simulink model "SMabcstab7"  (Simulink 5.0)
settings: Solver=ode45  StartTime=0.0  StopTime=6  MaxStep=2e-4  RelTol=1e-4
InitFcn:
  | smparamstab7
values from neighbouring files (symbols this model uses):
  Bm = 0.10    (= 0.1)    [IMabc2.m]    (also in imabcparam.m = 0.01; IMabcrun0.m = 0.01; IMabcrun1.m = 0.001; IMcur0.m = 1e-06)
  gam = 2*pi/3    (= 2.09439510239)    [IMabc2.m]    (also in IMabcf0.m; IMabcf1.m; imabcparam.m; IMabcrun0.m)
  H = 0.60    (= 0.6)    [IMabc2.m]    (also in IMcur0.m = 0.3; imdef0vec.m = 0.3; imdef1vec.m = 0.3; imdef2vec.m = 0.3)
  Lrr = [Lr   -Lm/2 -Lm/2    [IMabc2.m]    (also in IMabcf0.m = [Lr   -Lm1/2 -Lm1/2; IMabcf1.m = [Lr   -Lm1/2 -Lm1/2)
  R = str2num(get(h,'string'))    [acttrcalc1.m]    (also in IMabc2.m = diag([Rs Rs Rs Rr Rr Rr]); IMabcf0.m = diag([Rs Rs Rs Rr Rr Rr]); IMabcf1.m = diag([Rs Rs Rs Rr Rr Rr]); IMcurf0.m = diag([Rs Rs Rr Rr]))
  tc = abs(fco)    [im3phase.m]
  Vm = Vll*sqrt(2/3)    [imabcparam.m]
  wo = 2*pi*freq0    [calc0.m]    (also in IMabc2.m = 376.991118431; imabcparam.m = 376.991118431; IMabcrun0.m = 376.991118431; IMabcrun1.m = 376.991118431)
undefined symbols (not defined in the file or in its folder): ifo, L2, Labo, Laf, Lakd, Lakq, Lao, TL, to, vf
libraries: simulink x11

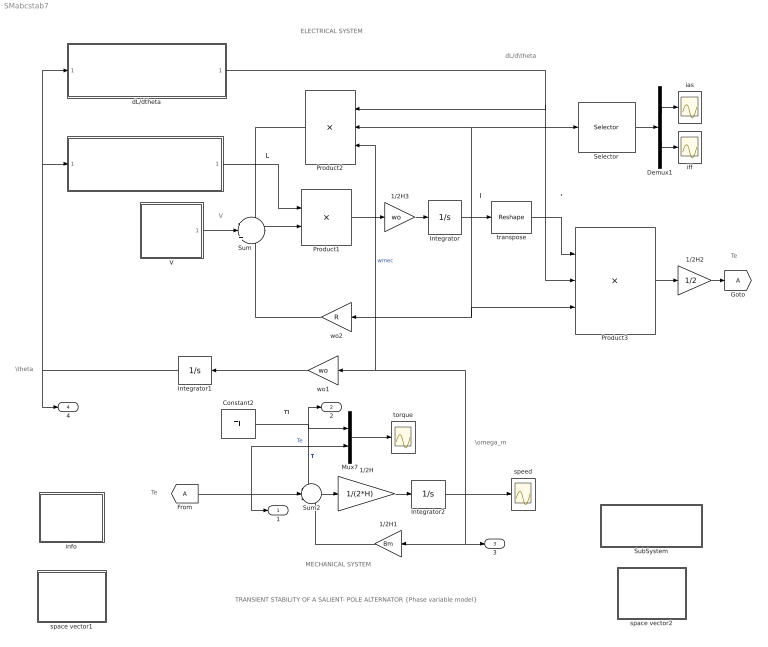
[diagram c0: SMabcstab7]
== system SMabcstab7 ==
  note: I
  note: I'
  note: MECHANICAL SYSTEM
  note: ELECTRICAL SYSTEM
  note: V
  note: TRANSIENT STABILITY OF A SALIENT- POLE ALTERNATOR {Phase variable model}
  note: L
  note: Te
  note: TL
  note: Te
  note: \theta
  note: \omega_m
  note: dL/d\theta
  1/2H : Gain  Gain=1/(2*H)
  1/2H1 : Gain  Orientation=left  Gain=Bm
  1/2H2 : Gain  Gain=1/2
  1/2H3 : Gain  Gain=wo
  Constant2 : Constant  Value=TL  VectorParams1D=off
  Demux1 : Demux  Outputs=2
  Integrator : Integrator  InitialCondition="[-0.3314    0.2780    0.0534  ifo 0 0 ]'"
  Integrator1 : Integrator  Orientation=left  InitialCondition=5.0571
  Integrator2 : Integrator  InitialCondition=1
  L : Subsystem
  Mux7 : Mux  Inputs=2
  Product1 : Product  Inputs=/*  Multiplication=Matrix(*)
  Product2 : Product  Orientation=left  Inputs=***  Multiplication=Matrix(*)
  Product3 : Product  Inputs=3  Multiplication=Matrix(*)  ShowAdditionalParam=on
  Selector : Selector  Elements=[1 4]  InputPortWidth=6
  SubSystem : Subsystem
  Sum : Sum  Inputs=-|+|-
  Sum2 : Sum  Inputs=-+-
  V : Subsystem
  dL/dtheta : Subsystem
  ias : Scope
  iff : Scope
  info : Subsystem
  space vector1 : Subsystem
  space vector2 : Subsystem
  speed : Scope
  torque : Scope
  transpose : simulink/Math Operations/Reshape  OutputDimensionality=Row vector  OutputDimensions=[1,6]
  wo1 : Gain  Orientation=left  Gain=wo
  wo2 : Gain  Orientation=left  Gain=R  Multiplication=Matrix(K*u)
  1 : Outport
  2 : Outport  Port=2
  3 : Outport  Port=3
  4 : Outport  Port=4
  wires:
  Product1/1 -> 1/2H3/1
  Sum/1 -> Product1/2
  transpose/1 -> Product3/1
  Product2/1 -> Sum/1
  dL/dtheta/1(dLdtheta) -> Product2/1, Product3/2
  Product3/1 -> 1/2H2/1
  Sum2/1 -> 1/2H/1
  1/2H/1 -> Integrator2/1
  1/2H1/1 -> Sum2/3
  Mux7/1 -> torque/1
  Constant2/1 -> Mux7/1, Sum2/1, 2/1  "TL"
  [A] -> Sum2/2, 1/1, Mux7/2  "Te"
  Integrator2/1 -> Product2/3, wo1/1, speed/1, 1/2H1/1, 3/1  "wmec"
  V/1(V) -> Sum/2
  Integrator1/1 -> dL/dtheta/1(theta1), L/1(theta), 4/1
  1/2H2/1 -> [A]
  L/1(L) -> Product1/1
  Integrator/1 -> transpose/1, Product2/2, Selector/1, Product3/3, wo2/1
  Selector/1 -> Demux1/1
  Demux1/2 -> iff/1
  Demux1/1 -> ias/1
  1/2H3/1 -> Integrator/1
  wo1/1 -> Integrator1/1
  wo2/1 -> Sum/3

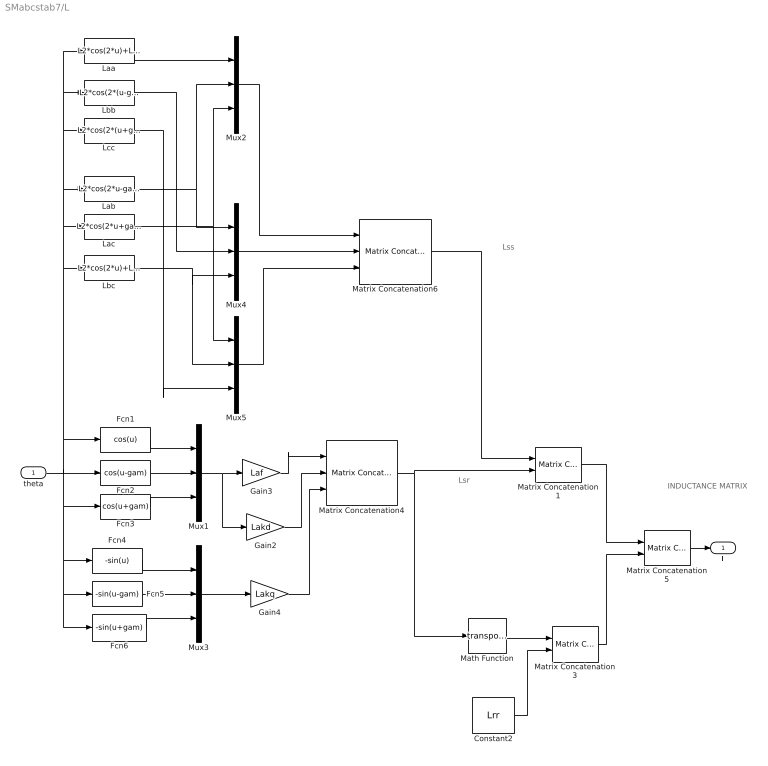
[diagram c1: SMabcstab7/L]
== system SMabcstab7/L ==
  note: INDUCTANCE MATRIX
  note: Lss
  note: Lsr
  theta : Inport
  Constant2 : Constant  Value=Lrr  VectorParams1D=off
  Fcn1 : Fcn  Expr=cos(u)
  Fcn2 : Fcn  Expr=cos(u-gam)
  Fcn3 : Fcn  Expr=cos(u+gam)
  Fcn4 : Fcn  Expr=-sin(u)
  Fcn5 : Fcn  Expr=-sin(u-gam)
  Fcn6 : Fcn  Expr=-sin(u+gam)
  Gain2 : Gain  Gain=Lakd
  Gain3 : Gain  Gain=Laf
  Gain4 : Gain  Gain=Lakq
  Laa : Fcn  Expr=L2*cos(2*u)+Lao
  Lab : Fcn  Expr=L2*cos(2*u-gam)+Labo
  Lac : Fcn  Expr=L2*cos(2*u+gam)+Labo
  Lbb : Fcn  Expr=L2*cos(2*(u-gam))+Lao
  Lbc : Fcn  Expr=L2*cos(2*u)+Labo
  Lcc : Fcn  Expr=L2*cos(2*(u+gam))+Lao
  Math Function : Math  Operator=transpose
  Matrix Concatenation1 : simulink/Math Operations/Matrix Concatenation  numInports=2  catMethod=Horizontal
  Matrix Concatenation3 : simulink/Math Operations/Matrix Concatenation  numInports=2  catMethod=Horizontal
  Matrix Concatenation4 : simulink/Math Operations/Matrix Concatenation  numInports=3  catMethod=Horizontal
  Matrix Concatenation5 : simulink/Math Operations/Matrix Concatenation  numInports=2  catMethod=Vertical
  Matrix Concatenation6 : simulink/Math Operations/Matrix Concatenation  numInports=3  catMethod=Horizontal
  Mux{1..5} (5 alike) : Mux  Inputs=3
  L : Outport
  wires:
  Matrix Concatenation5/1 -> L/1
  Matrix Concatenation4/1 -> Matrix Concatenation1/2, Math Function/1
  Mux1/1 -> Gain3/1, Gain2/1
  Matrix Concatenation1/1 -> Matrix Concatenation5/1
  Fcn3/1 -> Mux1/3
  Fcn2/1 -> Mux1/2
  Fcn1/1 -> Mux1/1
  theta/1 -> Fcn2/1, Fcn3/1, Fcn6/1, Fcn5/1, Fcn4/1, Fcn1/1, Laa/1, Lbb/1, Lcc/1, Lab/1, Lac/1, Lbc/1
  Gain3/1 -> Matrix Concatenation4/1
  Gain2/1 -> Matrix Concatenation4/2
  Fcn5/1 -> Mux3/2
  Fcn4/1 -> Mux3/1
  Fcn6/1 -> Mux3/3
  Mux3/1 -> Gain4/1
  Gain4/1 -> Matrix Concatenation4/3
  Math Function/1 -> Matrix Concatenation3/1
  Constant2/1 -> Matrix Concatenation3/2
  Matrix Concatenation3/1 -> Matrix Concatenation5/2
  Laa/1 -> Mux2/1
  Lbb/1 -> Mux4/2
  Lab/1 -> Mux2/2, Mux4/1
  Lac/1 -> Mux2/3, Mux5/1
  Lbc/1 -> Mux4/3, Mux5/2
  Lcc/1 -> Mux5/3
  Mux4/1 -> Matrix Concatenation6/2
  Mux2/1 -> Matrix Concatenation6/1
  Mux5/1 -> Matrix Concatenation6/3
  Matrix Concatenation6/1 -> Matrix Concatenation1/1

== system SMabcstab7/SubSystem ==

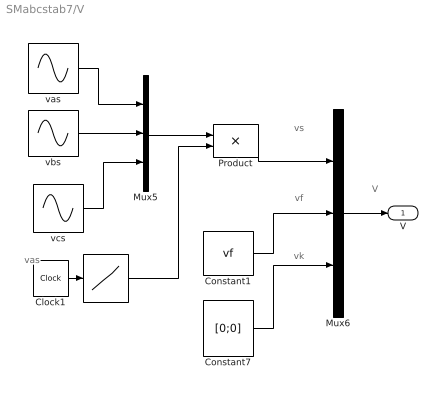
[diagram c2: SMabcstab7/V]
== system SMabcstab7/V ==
  note: V
  note: vas
  note: vs
  note: vf
  note: vk
  " " : Lookup  InputValues=[0 to to to+tc to+tc 10]  OutputValues="[1 1 0 0  1 1]"
  Clock1 : Clock
  Constant1 : Constant  Value=vf  VectorParams1D=off
  Constant7 : Constant  Value=[0;0]  VectorParams1D=off
  Mux5 : Mux  Inputs=3
  Mux6 : Mux  Inputs=3
  Product : Product
  vas : Sin  Amplitude=Vm  Frequency=wo  Phase=pi/2  SampleTime=0
  vbs : Sin  Amplitude=Vm  Frequency=wo  Phase=pi/2-gam  SampleTime=0
  vcs : Sin  Amplitude=Vm  Frequency=wo  Phase=pi/2+gam  SampleTime=0
  V : Outport
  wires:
  Mux6/1 -> V/1
  vbs/1 -> Mux5/2
  vas/1 -> Mux5/1
  vcs/1 -> Mux5/3
  Mux5/1 -> Product/1
  Clock1/1 -> " "/1
  " "/1 -> Product/2
  Product/1 -> Mux6/1
  Constant1/1 -> Mux6/2
  Constant7/1 -> Mux6/3

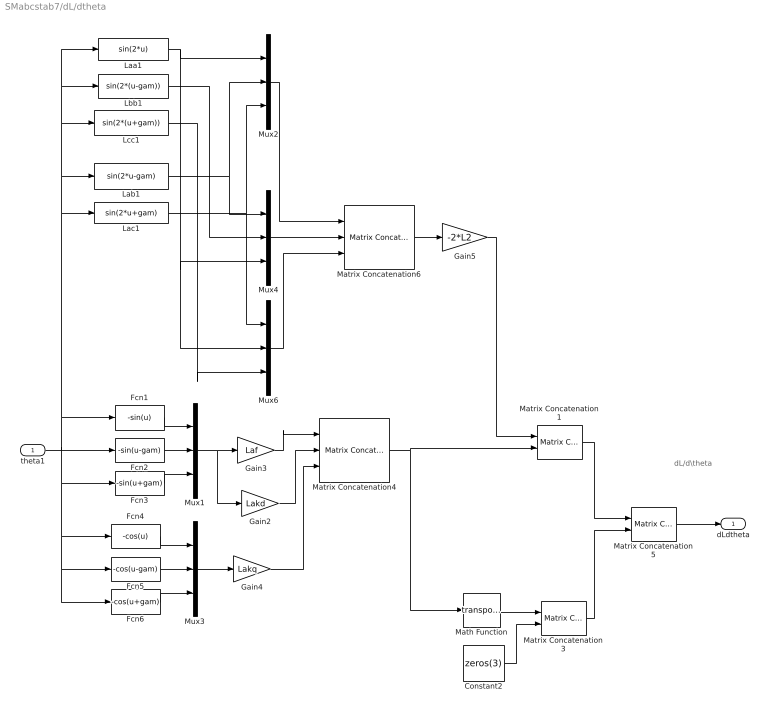
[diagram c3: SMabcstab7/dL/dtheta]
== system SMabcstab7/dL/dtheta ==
  note: dL/d\theta
  theta1 : Inport
  Constant2 : Constant  Value=zeros(3)  VectorParams1D=off
  Fcn1 : Fcn  Expr=-sin(u)
  Fcn2 : Fcn  Expr=-sin(u-gam)
  Fcn3 : Fcn  Expr=-sin(u+gam)
  Fcn4 : Fcn  Expr=-cos(u)
  Fcn5 : Fcn  Expr=-cos(u-gam)
  Fcn6 : Fcn  Expr=-cos(u+gam)
  Gain2 : Gain  Gain=Lakd
  Gain3 : Gain  Gain=Laf
  Gain4 : Gain  Gain=Lakq
  Gain5 : Gain  Gain=-2*L2
  Laa1 : Fcn  Expr=sin(2*u)
  Lab1 : Fcn  Expr=sin(2*u-gam)
  Lac1 : Fcn  Expr=sin(2*u+gam)
  Lbb1 : Fcn  Expr=sin(2*(u-gam))
  Lcc1 : Fcn  Expr=sin(2*(u+gam))
  Math Function : Math  Operator=transpose
  Matrix Concatenation1 : simulink/Math Operations/Matrix Concatenation  numInports=2  catMethod=Horizontal
  Matrix Concatenation3 : simulink/Math Operations/Matrix Concatenation  numInports=2  catMethod=Horizontal
  Matrix Concatenation4 : simulink/Math Operations/Matrix Concatenation  numInports=3  catMethod=Horizontal
  Matrix Concatenation5 : simulink/Math Operations/Matrix Concatenation  numInports=2  catMethod=Vertical
  Matrix Concatenation6 : simulink/Math Operations/Matrix Concatenation  numInports=3  catMethod=Horizontal
  Mux{1..4,6} (5 alike) : Mux  Inputs=3
  dLdtheta : Outport
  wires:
  Matrix Concatenation5/1 -> dLdtheta/1
  Matrix Concatenation4/1 -> Matrix Concatenation1/2, Math Function/1
  Mux1/1 -> Gain3/1, Gain2/1
  Matrix Concatenation1/1 -> Matrix Concatenation5/1
  Fcn3/1 -> Mux1/3
  Fcn2/1 -> Mux1/2
  Fcn1/1 -> Mux1/1
  theta1/1 -> Fcn2/1, Fcn3/1, Fcn6/1, Fcn5/1, Fcn4/1, Fcn1/1, Laa1/1, Lbb1/1, Lcc1/1, Lab1/1, Lac1/1
  Gain3/1 -> Matrix Concatenation4/1
  Gain2/1 -> Matrix Concatenation4/2
  Fcn5/1 -> Mux3/2
  Fcn4/1 -> Mux3/1
  Fcn6/1 -> Mux3/3
  Mux3/1 -> Gain4/1
  Gain4/1 -> Matrix Concatenation4/3
  Math Function/1 -> Matrix Concatenation3/1
  Constant2/1 -> Matrix Concatenation3/2
  Matrix Concatenation3/1 -> Matrix Concatenation5/2
  Laa1/1 -> Mux2/1, Mux4/3, Mux6/2
  Lbb1/1 -> Mux4/2
  Lab1/1 -> Mux2/2, Mux4/1
  Lac1/1 -> Mux2/3, Mux6/1
  Lcc1/1 -> Mux6/3
  Mux4/1 -> Matrix Concatenation6/2
  Mux2/1 -> Matrix Concatenation6/1
  Mux6/1 -> Matrix Concatenation6/3
  Matrix Concatenation6/1 -> Gain5/1
  Gain5/1 -> Matrix Concatenation1/1

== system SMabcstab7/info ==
  note: SYNCHRONOUS MACHINE STABILITY SALIENT POLE ROTOR (Phase variable model)
  note: A salient pole synchronous generator is running in steady state under load when a three phase short occurs at the terminals . A few cycles later, the fault is cleared. The dynamic equations are expressed in matrix form in terms the phase variables, namely the stator currents ias, ibs, ics; the rotor field current iff; the d-axis and q-axis damper currents idk and iqk; the anglar speed wm; and the displacement angle theta between stator as-axis and rotor direct axis. Torque, speed and current responses are plotted.The torque angle is also shown. A Matlab script file for the identical system operation is given in the file >.

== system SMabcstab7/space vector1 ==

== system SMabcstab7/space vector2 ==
